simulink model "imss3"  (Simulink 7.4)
settings: Solver=ode45  StartTime=0.0  StopTime=0  MaxStep=3

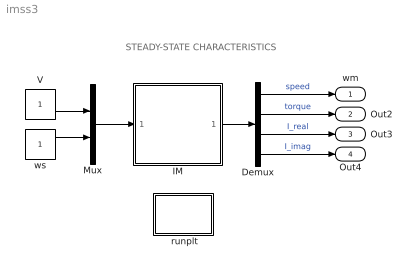
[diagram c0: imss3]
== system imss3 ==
  note: STEADY-STATE CHARACTERISTICS
  " runplt" : Subsystem
  Demux : Demux
  IM : Subsystem  mask{Rs=0.01, Rr=0.02, Lsl=0.1, Lrl=0.1, Lm=4.5, wm=[0:0.01:2.0]}
      mask prompts: Rs "Stator resistance [pu]"; Rr "Rotor Resistance [pu]"; Lsl "Stator leakage inductance [pu]"; Lrl "Rotor leakage inductance [pu]"; Lm "Magnetizing inductance [pu]"; wm "Speed range ]pu]"
  Mux : Mux  Inputs=2
  V : Constant  OutDataType=sfix(16)  OutScaling=2^0
  ws : Constant  OutDataType=sfix(16)  OutScaling=2^0
  wm : Outport
  Out2 : Outport  Port=2
  Out3 : Outport  Port=3
  Out4 : Outport  Port=4
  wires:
  ws/1 -> Mux/2
  V/1 -> Mux/1
  Demux/3 -> Out3/1  "I_real"
  Demux/2 -> Out2/1  "torque"
  Demux/1 -> wm/1  "speed"
  IM/1(Out1) -> Demux/1
  Mux/1 -> IM/1(In1)
  Demux/4 -> Out4/1  "I_imag"

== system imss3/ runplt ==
  note: This demo develops the steady-state characteristics of an induction motor
  note: Double click the block to view torque-speed and current-speed curves and the current circle diagram
  note: First start the simulation, then

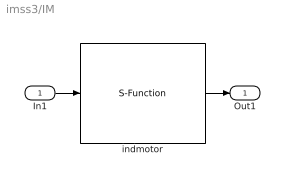
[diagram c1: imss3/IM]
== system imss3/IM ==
  In1 : Inport  OutDataType=sfix(16)  OutScaling=2^0
  indmotor : S-Function  FunctionName=imssmod3  Parameters=Rs,Rr,Lsl,Lrl,Lm,wm  EnableBusSupport=off
  Out1 : Outport
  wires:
  In1/1 -> indmotor/1
  indmotor/1 -> Out1/1
